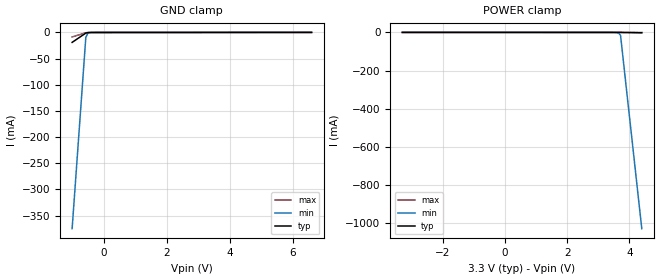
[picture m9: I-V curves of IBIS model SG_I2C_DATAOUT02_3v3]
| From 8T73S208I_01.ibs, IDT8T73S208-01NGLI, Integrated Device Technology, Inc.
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[Model] SG_I2C_DATAOUT02_3v3
Model_type   Input
Polarity   Non-Inverting
Vinl = 0.8V
Vinh = 2.0V
|   typ   min   max
C_comp   2pF   1.5pF   2.5pF
|   typ   min   max
[Voltage range]   3.3V   3.135V   3.465V
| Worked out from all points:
|   GND clamp passes 1 mA (typ) near -0.54 V on its own axis
[GND_clamp]
|Voltage   I (typ)   I (min)   I (max)
-999mV    -18.98mA   -375.1mA   -8.614mA
-564.6mV  -1.3mA     -9.505mA   -655.5uA
-502.5mV  -459.7uA   -1.83mA    -187.8uA
-316.4mV  -73.13uA   -84.35uA   -70.18uA
6.6V      65.18uA    70.68uA    58.13uA
[Power_clamp]
|Voltage   I (typ)   I (min)   I (max)
-3.3V     65.18uA    67.32uA    61.19uA
3.655V    -78.59uA   -2.855mA   -67.78uA
3.717V    -117.3uA   -15.95mA   -68.94uA
4.4V      -2.165mA   -1.028A    -82.17uA
